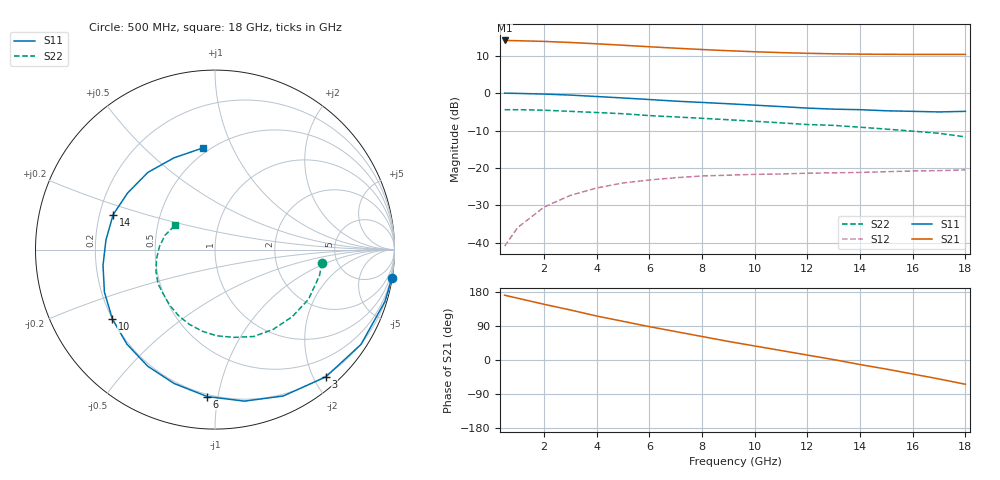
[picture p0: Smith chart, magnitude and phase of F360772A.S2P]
!ATF-36077
!S AND NOISE PARAMETERS at Vds=1.5V  Id=10mA.  LAST UPDATED 06-27-94
# ghz s ma r 50
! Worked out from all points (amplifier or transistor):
!   19 points, 500 MHz to 18 GHz, reference 50 ohm
!   highest |S21| = 14.1 dB at 500 MHz (marker M1)
!   |S21| within 3 dB of that: start of sweep to 9.92 GHz
!   unconditionally stable (mu >= 1): 14.84 GHz to end of sweep
!   at 3 GHz: K = 0.24, MSG = 20.4 dB, |S12| = -27.3 dB
!   at 9 GHz: K = 0.69, MSG = 16.6 dB, |S12| = -21.9 dB
!   at 18 GHz: K = 1.03, MAG = 14.4 dB, |S12| = -20.5 dB
!   lowest NFmin = 0.30 dB at 1 GHz
!   S11 on the Smith chart (normalised r, x): 500 MHz: 0, -13; 3 GHz: 0.18, -2.18; 6 GHz: 0.19, -0.93; 10 GHz: 0.20, -0.29; 14 GHz: 0.26, +0.16; 18 GHz: 0.46, +0.77
0.5  0.998 -9.0  5.05 171.0  0.009 83.0  0.6 -7.0
1  0.99 -17.0  5.01 163.0  0.016 78.0  0.6 -14.0
2  0.97 -33.0  4.904 147.0  0.03 66.0  0.59 -28.0
3  0.94 -49.0  4.745 132.0  0.043 54.0  0.57 -41.0
4  0.9 -65.0  4.556 116.0  0.054 43.0  0.55 -54.0
5  0.86 -79.0  4.357 102.0  0.063 33.0  0.53 -66.0
6  0.82 -93.0  4.162 88.0  0.069 24.0  0.5 -78.0
7  0.78 -107.0  3.981 75.0  0.074 16.0  0.48 -89.0
8  0.75 -120.0  3.82 62.0  0.078 8.0  0.46 -99.0
9  0.72 -133.0  3.682 49.0  0.08 1.0  0.44 -109.0
10  0.69 -146.0  3.566 37.0  0.082 -6.0  0.42 -119.0
11  0.66 -159.0  3.473 25.0  0.083 -13.0  0.4 -129.0
12  0.63 -172.0  3.401 13.0  0.085 -19.0  0.38 -139.0
13  0.61 175.0  3.349 1.0  0.086 -25.0  0.37 -149.0
14  0.6 161.0  3.315 -12.0  0.087 -32.0  0.35 -160.0
15  0.58 147.0  3.296 -24.0  0.089 -39.0  0.33 -171.0
16  0.57 131.0  3.289 -37.0  0.091 -47.0  0.31 177.0
17  0.56 114.0  3.289 -50.0  0.092 -55.0  0.29 164.0
18  0.57 97.0  3.291 -64.0  0.094 -65.0  0.26 148.0
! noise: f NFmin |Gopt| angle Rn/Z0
1  0.3  0.95  12  0.4
2  0.3  0.9  25  0.2
4  0.3  0.81  51  0.17
6  0.3  0.73  76  0.13
8  0.37  0.66  102  0.09
10  0.44  0.6  129  0.05
12  0.5  0.54  156  0.03
14  0.56  0.48  -174  0.02
16  0.61  0.43  -139  0.05
18  0.65  0.39  -100  0.09
